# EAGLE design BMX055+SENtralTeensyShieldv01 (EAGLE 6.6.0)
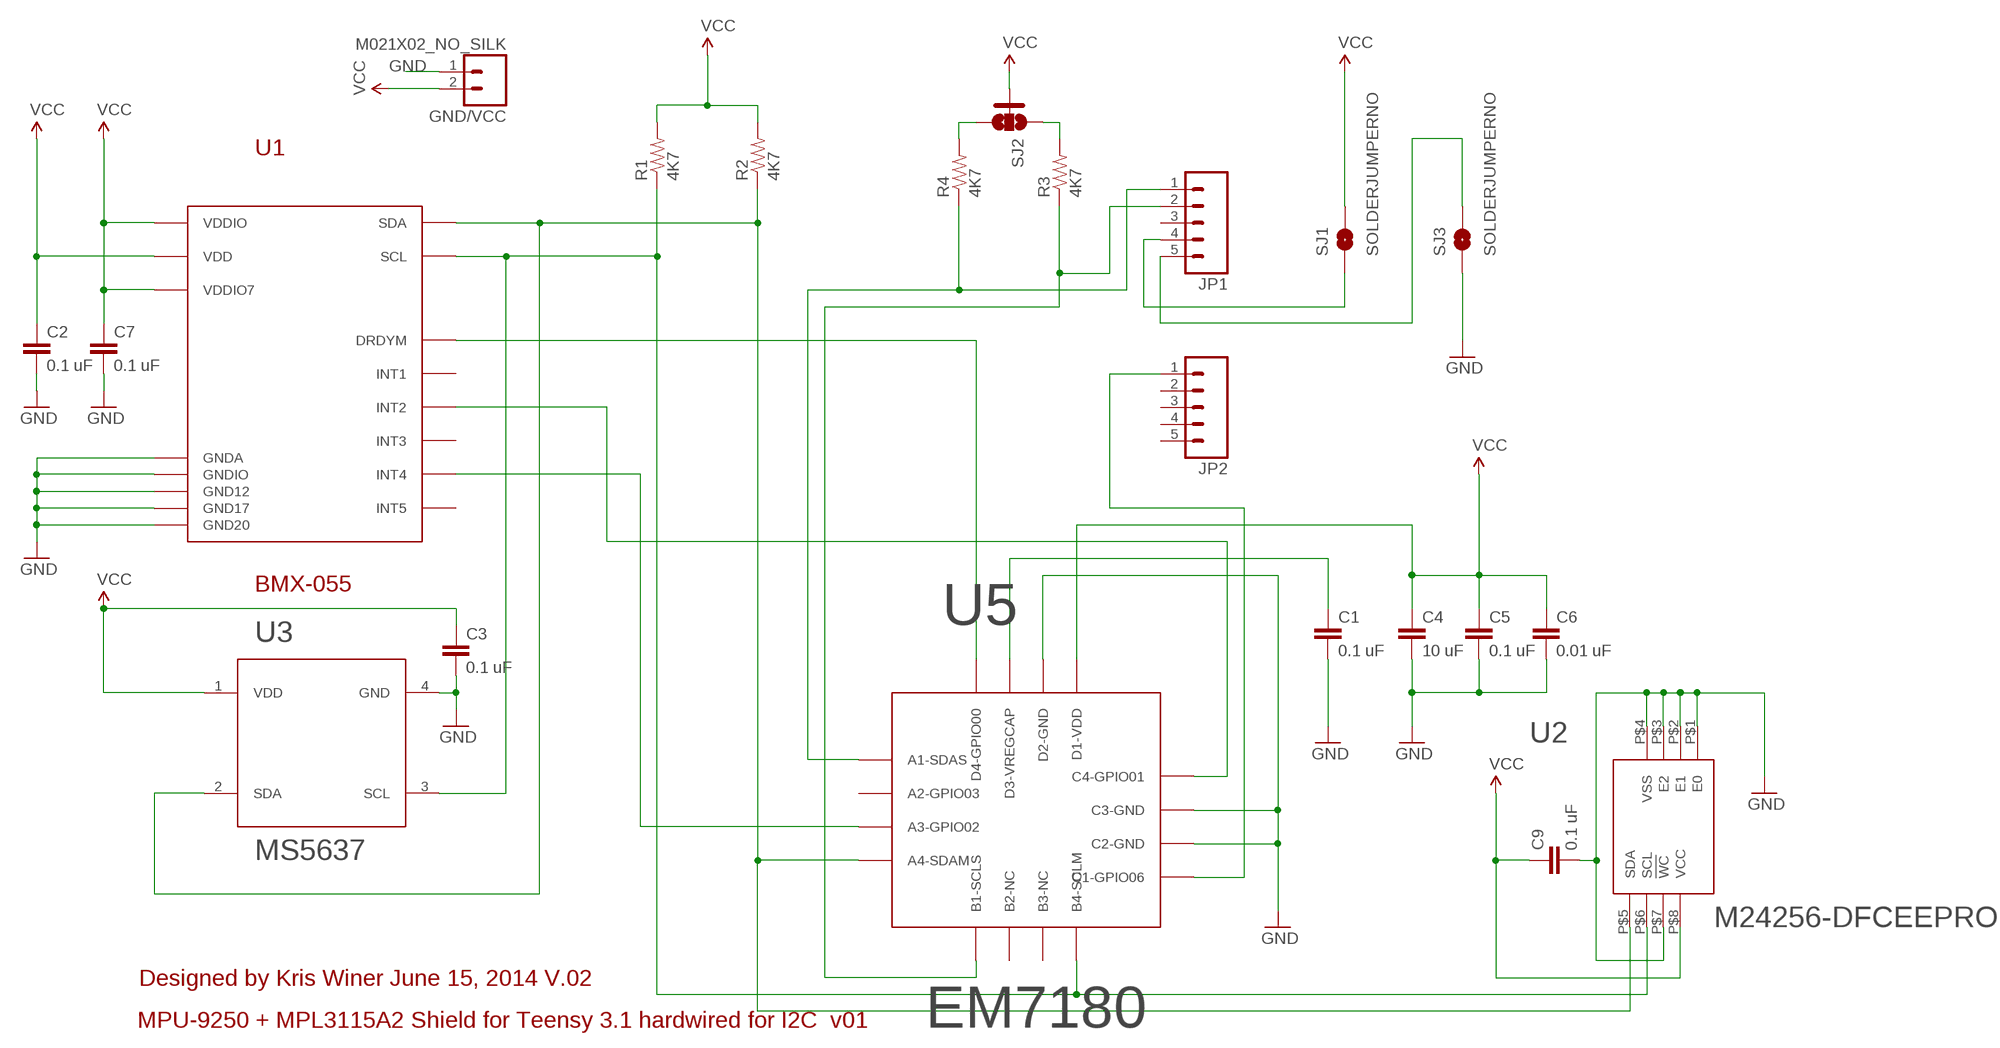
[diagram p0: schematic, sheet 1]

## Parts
C1  0.1 uF  CAP0402-CAP  [0402-CAP]
C2  0.1 uF  CAP0402-CAP  [0402-CAP]
C3  0.1 uF  CAP0402-CAP  [0402-CAP]
C4  10 uF  CAP0402-CAP  [0402-CAP]
C5  0.1 uF  CAP0402-CAP  [0402-CAP]
C6  0.01 uF  CAP0402-CAP  [0402-CAP]
C7  0.1 uF  CAP0402-CAP  [0402-CAP]
C9  0.1 uF  CAP0402-CAP  [0402-CAP]
GND/VCC  M021X02_NO_SILK  [1X02_NO_SILK]
JP1  M05NO_SILK  [1X05_NO_SILK]
JP2  M05NO_SILK  [1X05_NO_SILK]
R1  4K7  RESISTOR0402-RES  [0402-RES]
R2  4K7  RESISTOR0402-RES  [0402-RES]
R3  4K7  RESISTOR0402-RES  [0402-RES]
R4  4K7  RESISTOR0402-RES  [0402-RES]
SJ1  SOLDERJUMPERNO  [SJ_2S-NO]
SJ2  SOLDERJUMPER_2WAYS  [SJ_3]
SJ3  SOLDERJUMPERNO  [SJ_2S-NO]
U1  BMX-055  [BMX-055]
U2  M24256-DFCEEPROM  [UFDFPN8]
U3  MS5637  [MS5637QFN-4]
U5  EM7180  [WL-CSP16]

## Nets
GND: C1.2 C2.2 C3.2 C4.2 C5.2 C6.2 C7.2 C9.2 GND/VCC.1 SJ3.1 U1.4(GNDA) U1.6(GNDIO) U1.12(GND12) U1.17(GND17) U1.20(GND20) U2.P$1(E0) U2.P$2(E1) U2.P$3(E2) U2.P$4(VSS) U2.P$7(!WC) U3.4(GND) U5.P$10(C2-GND) U5.P$11(C3-GND) U5.P$14(D2-GND)
N$1: U1.2(DRDYM) U5.P$16(D4-GPIO00)
N$2: U1.1(INT2) U5.P$12(C4-GPIO01)
N$3: U1.15(INT4) U5.P$3(A3-GPIO02)
N$4: JP2.1 U5.P$9(C1-GPIO06)
N$5: R4.2 SJ2.3
N$6: R3.2 SJ2.1
N$7: JP1.4 SJ1.1
N$8: JP1.5 SJ3.2
N$9: C1.1 U5.P$15(D3-VREGCAP)
SCL: R1.1 U1.9(SCL) U2.P$6(SCL) U3.3(SCL) U5.P$8(B4-SCLM)
SCL1: JP1.1 R4.1 U5.P$1(A1-SDAS)
SDA: R2.1 U1.11(SDA) U2.P$5(SDA) U3.2(SDA) U5.P$4(A4-SDAM)
SDA1: JP1.2 R3.1 U5.P$5(B1-SCLS)
VCC: C2.1 C3.1 C4.1 C5.1 C6.1 C7.1 C9.1 GND/VCC.2 R1.2 R2.2 SJ1.2 SJ2.2 U1.3(VDD) U1.7(VDDIO7) U1.13(VDDIO) U2.P$8(VCC) U3.1(VDD) U5.P$13(D1-VDD)
Unconnected: JP1.3 JP2.2 JP2.3 JP2.4 JP2.5 U1.10(INT5) U1.14(INT3) U1.19(INT1) U5.P$2(A2-GPIO03) U5.P$6(B2-NC) U5.P$7(B3-NC)

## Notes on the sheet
- Designed by Kris Winer June 15, 2014 V.02
- MPU-9250 + MPL3115A2 Shield for Teensy 3.1 hardwired for I2C  v01

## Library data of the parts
C1-C7 C9 = SparkFun-Capacitors:CAP: Capacitor
GND/VCC = SparkFun-Connectors:M02: Standard 2-pin 0.1" header. Use with
JP1 JP2 = SparkFun-Connectors:M05: Header 5 Standard 5-pin 0.1" header. Use with straight break away headers (SKU : PRT-00116), right angle break away headers (PRT-00553), swiss pins (PRT-00743), machine pins (PRT-00117), and female headers (PRT-00115). Molex polarized connector foot print use with SKU : PRT-08230 with associated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
R1-R4 = SparkFun-Passives:RESISTOR: Resistor
SJ1 SJ3 = SparkFun-Retired:SOLDERJUMPER: Solder Jumper
SJ2 = SparkFun-Passives:SOLDERJUMPER_2WAY: Solder Jumper 2 way solder jumper
U1 = SparkFun-DiscreteSemi:BMX-055: Device symbol for BMX-055 9-axis sensor in LGA-20 package.
U2 = SparkFun-DigitalIC:M24256-DFCEEPROM: M24256-DFC I2C EEPROM for use with EM7180 SENtral sensor fusion hub
U3 = SparkFun-DiscreteSemi:MS5637: MS5637 I2C pressure sensor in QFN-4 package by Measurement Specialties
U5 = SparkFun-DigitalIC:EM7180: WL-CSP19 package for the EM7180 SENtral sensor fusion hub

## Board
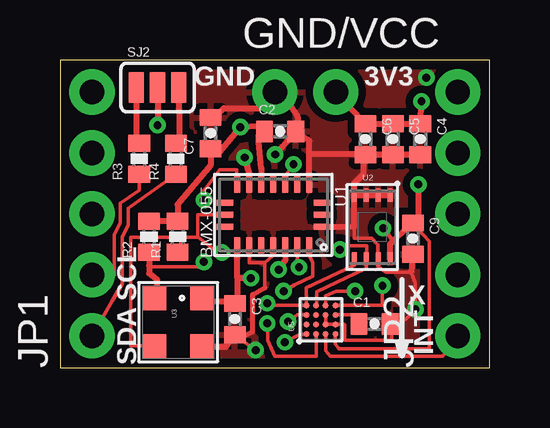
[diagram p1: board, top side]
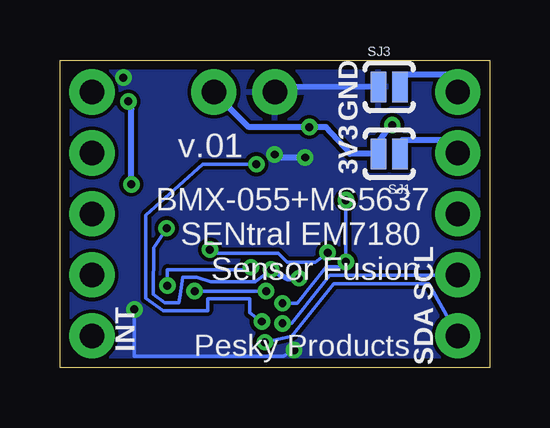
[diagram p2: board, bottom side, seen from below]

Size 17.91 x 12.83 mm. Coordinates in mm from the lower left corner, seen from the top.
Outline: 0,0 17.91,0 17.91,12.83 0,12.83 0,0
Copper layers (1*16): Top 0.0356mm / dielectric 1.5011mm / Bottom 0.0356mm
Design rules "OSHPark *": minimum track width 6mil, minimum drill 13mil, track to track 6mil, track to pad 6mil, pad to pad 6mil, via to via 6mil, smd to smd 6mil, copper to edge 15mil, drill to drill 6mil, minimum pad ring 7mil, minimum via ring 7mil, stop-mask expansion 3mil, vias tented up to drill 20mil, thermal gap 10mil

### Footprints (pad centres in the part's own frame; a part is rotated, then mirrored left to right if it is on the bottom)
0402-CAP = smd 0.7 x 0.9: 1 -0.65,0; 2 0.65,0
1X02_NO_SILK = drill 1.016 pad 1.88: 1 0,0; 2 2.54,0
1X05_NO_SILK = drill 1.016 pad 1.88: 1 0,0; 2 2.54,0; 3 5.08,0; 4 7.62,0; 5 10.16,0
0402-RES = smd 0.7 x 0.9: 1 -0.65,0; 2 0.65,0
SJ_2S-NO = smd 0.635 x 1.27: 1 -0.45,0; 2 0.45,0
SJ_3 = smd 0.635 x 1.27: 1 -0.889,0; 2 0,0; 3 0.889,0
BMX-055 = smd 0.675 x 0.25: 1 1.262,1.5; 2 1.262,1; 3 1.262,0.5; 4 1.262,0; 5 1.262,-0.5; 6 1.262,-1; 7 1.262,-1.5; 11 -1.262,-1.5; 12 -1.262,-1; 13 -1.262,-0.5; 14 -1.262,0; 15 -1.262,0.5; 16 -1.262,1; 17 -1.262,1.5 | smd 0.25 x 0.675: 8 0.5,-2.013; 9 0,-2.013; 10 -0.5,-2.013; 18 -0.5,2.013; 19 0,2.013; 20 0.5,2.013
UFDFPN8 = smd 0.2 x 0.55: P$1 0.75,1.325; P$2 0.25,1.325; P$3 -0.25,1.325; P$4 -0.75,1.325; P$5 -0.75,-1.325; P$6 -0.25,-1.325; P$7 0.25,-1.325; P$8 0.75,-1.325
MS5637QFN-4 = smd 1 x 1: 1 -1,1; 2 -1,-1; 3 1,-1; 4 1,1
WL-CSP16 = smd 0.24 x 0.24: P$1 -0.6,0.6; P$2 -0.2,0.6; P$3 0.2,0.6; P$4 0.6,0.6; P$5 -0.6,0.2; P$6 -0.2,0.2; P$7 0.2,0.2; P$8 0.6,0.2; P$9 -0.6,-0.2; P$10 -0.2,-0.2; P$11 0.2,-0.2; P$12 0.6,-0.2; P$13 -0.6,-0.6; P$14 -0.2,-0.6; P$15 0.2,-0.6; P$16 0.6,-0.6

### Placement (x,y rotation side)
C1  13.11,1.83 0 top
C2  9.17,9.86 0 top
C3  7.29,2.03 270 top
C4  15.01,9.53 270 top
C5  13.87,9.53 270 top
C6  12.73,9.53 270 top
C7  6.27,9.78 90 top
C9  14.71,5.38 270 top
GND/VCC  8.95,11.49 0 top
JP1  1.33,1.33 90 top
JP2  16.57,1.33 90 top
R1  4.9,5.46 90 top
R2  3.71,5.46 90 top
R3  3.3,8.71 90 top
R4  4.83,8.71 90 top
SJ1  4.19,8.92 180 bottom
SJ2  4.06,11.68 0 top
SJ3  4.19,11.71 0 bottom
U1  8.89,6.38 270 top
U2  13,5.87 0 top
U3  4.93,1.91 270 top
U5  10.87,2.01 90 top

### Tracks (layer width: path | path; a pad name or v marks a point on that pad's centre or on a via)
GND  (via drill 0.33)
  Top 0.152: U1.4 8.89,4.7 8.53,4.37 | 12.26,5.89 12.26,5.39 13,5.39 13.23,5.13 13.23,4.56 U2.P$7 13.26,4.18 13.61,3.99 14.63,3.99 14.81,3.53 v14.81,2.44 14.4,2.03 C1.2 13.82,1.97 13.82,1.14 11.89,1.14 11.86,1.22 11.86,1.8 11.83,1.81 U5.P$14 U5.P$10 U5.P$11 | 7.42,1.19 C3.2 7.87,0.95 8,0.86 v8.15,0.74 | U1.6 7.89,4.37 8.53,4.37 | 8.53,3.33 8.53,4.37
  Top 0.203: 7.42,1.19 8.03,1.5 8.03,3.05 8.53,3.33
  Top 0.254: C4.2 C5.2 C6.2 | C6.2 12.68,8.89 10.41,8.89 10.39,8.87 | C7.2 6.35,10.34 6.83,10.82 8.28,10.82 GND/VCC.1 9.21,11.49 9.91,10.46 9.91,9.82 C2.2 | U2.P$1 U2.P$2 U2.P$3 U2.P$4 | U2.P$4 12.26,7.68 12.65,8.08 12.65,8.8 C6.2 | U3.4 6.51,0.87 6.91,0.87 C3.2 | U1.12 7.89,8.11 v7.7,8.76 | v8.97,8.89 9.46,9.45 9.72,9.78 C2.2 | U1.20 11.72,5.88 12.26,5.89 U2.P$4 | U1.17 10.39,8.87 | 10.39,8.87 10.39,9.46 10.11,9.64 C2.2 | C9.2 14.63,3.99
  Bottom 0.152: v14.81,2.44 14.81,0.48 8.61,0.48 v8.15,0.74
  Bottom 0.254: 8.89,11.43 GND/VCC.1 8.76,11.68 SJ3.1 | v7.7,8.76 8.81,8.76 v8.97,8.89
  other vias: 15.27,12.09
  pour Bottom: 0.03,12.83 0.03,-0.03 17.96,-0.03 17.96,12.8 0.05,12.8
  pour Top (isolate 0.305): 0.03,12.83 -0.03,12.83 -0.03,0 3.28,0 3.28,3.43 6.55,3.43 6.55,-0.03 17.96,-0.03 18.01,-0.03 18.01,12.83 0.1,12.83
N$1  (via drill 0.33)
  Top 0.152: U5.P$16 13.43,2.61 13.44,2.92 v13.44,3.43 | U1.2 9.89,4.3 v9.96,4.19
  Bottom 0.152: v13.44,3.43 13.44,4.09 10.06,4.09 v9.96,4.19
N$2  (via drill 0.33)
  Top 0.152: U5.P$12 11.07,2.79 11.07,3 11.51,3.2 v12.29,3.2 | U1.1 10.39,4.67 10.54,4.39 10.54,3.81 9.78,3.45 v9.32,3.2
  Bottom 0.152: v9.32,3.2 v12.29,3.2
N$3  (via drill 0.33)
  Top 0.152: U1.15 9.39,7.99 v9.73,8.48 | U5.P$3 9.88,2.21 v9.5,1.93
  Bottom 0.152: v9.73,8.48 11.96,8.48 14.33,6.35 14.33,2.9 13.61,2.39 11.76,2.39 11.76,2.87 10.01,2.87 10.01,2.29 v9.5,1.93
N$4
  Top 0.152: U5.P$9 11.07,0.71 11.25,0.48 15.95,0.48 JP2.1
N$5
  Top 0.254: SJ2.3 4.98,9.54 R4.2
N$6
  Top 0.254: SJ2.1 3.17,9.49 R3.2
N$7
  Bottom 0.152: 3.76,9.04 SJ1.1
  Bottom 0.254: JP1.4 1.43,9.47 3.68,9.47 3.79,9.09 3.76,9.04
N$8
  Bottom 0.254: JP1.5 1.4,12.22 3.68,12.22 SJ3.2
N$9
  Top 0.152: U5.P$15 12.21,2.21 C1.1
SCL  (via drill 0.33)
  Top 0.152: U1.9 5.74,6.38 5.74,5.44 | R1.1 5,4.7 5.04,4.89 | 5.04,4.89 5,5.44 | 5.05,5.44 2.95,5.44 2.95,0.91 3.92,0.91 | 5.74,5.44 5.05,5.44 | 5.05,5.44 5.04,4.89 | v6.76,4.8 6.6,4.8 5.77,5.44 5.74,5.44 | U5.P$8 10.69,2.63 10.69,3.17 12.75,4.14 U2.P$6 12.78,4.56 12.78,5.08 11.79,5.08 v11.66,4.93
  Top 0.254: 3.92,0.91 U3.3
  Bottom 0.152: v11.66,4.93 11.56,4.78 8.81,4.78 8.43,4.39 7.26,4.39 6.93,4.65 v6.76,4.8
SCL1  (via drill 0.33)
  Top 0.152: R4.1 4.51,7.83 2.85,6.66 2.85,5.97 2.59,5.44 2.59,3.5 2.18,2.79 JP1.1 | v9.37,1.07 10.01,1.4 U5.P$1
  Bottom 0.152: JP1.1 1.33,1.36 2.54,3.5 6.5,3.5 8.26,1.32 v9.37,1.07
SDA  (via drill 0.33)
  Top 0.152: U1.11 7.39,7.98 7.37,8.26 6.66,8.26 6.07,7.49 5.99,7.39 v5.99,6.99 | v5.99,4.42 5.99,4.22 3.76,4.22 3.71,4.27 | U2.P$5 12.27,4.27 10.26,3.33 10.26,2.69 U5.P$4 8.76,2.61 v8.64,2.69
  Top 0.254: R2.1 3.71,4.27 3.71,3.94 4.04,3.68 4.04,3.07 U3.2
  Bottom 0.152: v5.99,6.99 v5.99,4.42 5.99,4.22 6.81,4.22 8.03,2.69 v8.64,2.69
SDA1  (via drill 0.33)
  Top 0.152: R3.1 3.3,7.39 2.52,6.86 2.52,6.04 2.26,5.54 2.26,3.86 JP1.2 | v8.64,1.85 8.66,1.14 8.94,0.48 10.67,0.48 10.67,1.2 U5.P$5
  Bottom 0.152: JP1.2 1.44,3.85 6.67,3.85 8.26,1.85 v8.64,1.85
VCC  (via drill 0.33)
  Top 0.152: U5.P$13 11.47,1 11.61,0.79 15.39,0.79 15.39,5.27 C9.1 | 7.39,2.76 C3.1 | v13.46,5.82 13.54,5.79 13.87,5.28
  Top 0.254: GND/VCC.2 11.51,11.49 C6.1 C5.1 C4.1 15.02,11.1 v15.06,11.1 | U1.13 8.39,8.27 8.39,8.31 8.28,9.4 | R2.2 R1.2 4.9,6.81 6.27,8.43 C7.1 6.56,8.9 v7.52,10.03 8.29,10.06 8.28,9.4 | 8.28,9.4 8.39,9.68 C2.1 | 7.39,3.74 7.39,4.58 U1.7 | U3.1 6.26,2.77 7.23,2.77 C3.1 | SJ2.2 v4.06,10.11 | U1.3 9.39,4.5 v9.11,4.1 | v7.95,3.73 7.39,3.73 7.39,3.74 | 7.39,3.74 7.39,2.76 | v14.94,7.64 14.94,6.34 C9.1 13.87,5.28 13.76,5.16 U2.P$8
  Bottom 0.152: 4.67,9.02 SJ1.2 | v9.11,4.1 9.78,3.58 11.63,3.58 12.22,3.79 12.8,3.79 12.9,3.05 12.95,2.72 13.54,2.72 14.02,3.07 13.99,5 v13.46,5.82
  Bottom 0.254: SJ1.2 5.82,8.91 6.83,10.03 v7.52,10.03 10.03,10.03 GND/VCC.2 | v14.94,7.64 14.94,10.79 v15.06,11.1 | v4.06,10.11 4.06,10.21 4.67,9.37 4.67,9.02 | v9.11,4.1 8.46,3.73 v7.95,3.73

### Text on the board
tPlace: GND | 3V3 | SCL | X | INT | SDA
bPlace: GND | 3V3 | v.01 | BMX-055+MS5637 / SENtral EM7180 / Sensor Fusion | SCL | SDA | INT | Pesky Products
